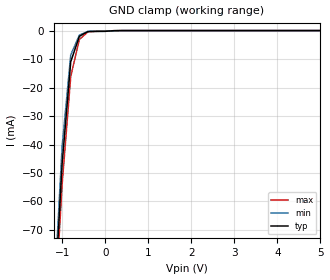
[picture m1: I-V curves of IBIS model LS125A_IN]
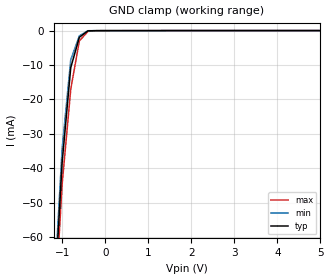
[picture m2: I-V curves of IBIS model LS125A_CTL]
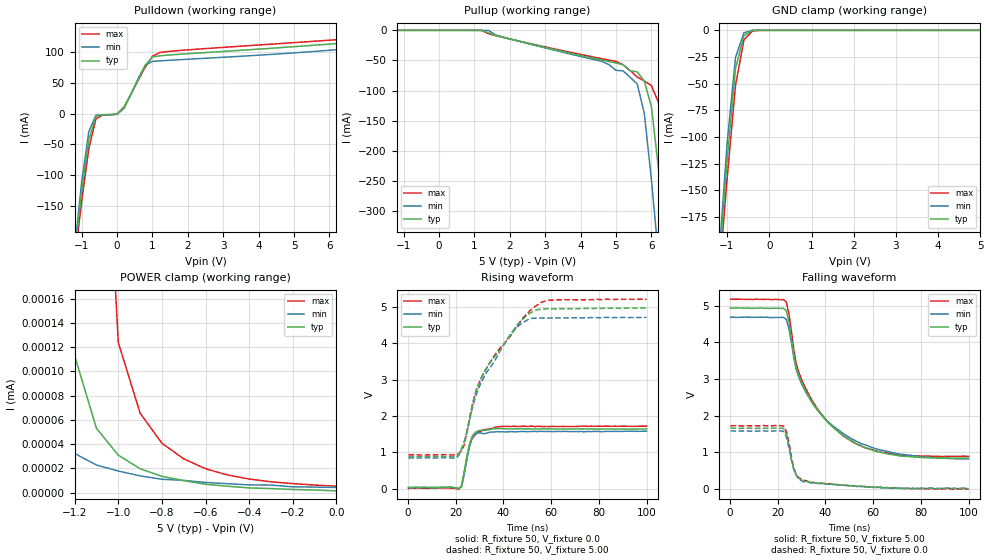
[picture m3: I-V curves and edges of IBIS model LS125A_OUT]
|   TEXAS INSTRUMENTS INCORPORATED
|   Standard Linear and Logic Group
|   IBIS Model of SN74LS125A
|   QUADRUPLE BUS BUFFERS WITH THREE-STATE OUTPUTS
|   SOIC 14-pin(D), SOP 14-pin(NS), PDIP 14-pin(N)
[IBIS Ver]   3.1
[Comment Char]  |_char
[File Name]   sn74ls125a.ibs
[File Rev]   1.1
[Date]   JULY 9, 2004
[Source]   File originated at Texas Instruments, Inc.
[Notes]   - FILE REV HISTORY
   - 1.1 Release IBIS file on 07/10/04
   - All test data contained in this file are derived from
   actual measurements.
   - The measurements used D package.
[Disclaimer] Property of Texas Instruments Incorporated.  Unauthorized
   reproduction and/or distribution is strictly prohibited.
   This product is protected under copyright law.
   Created 2000, (C) Copyright 2000, Texas Instruments Inc.,
   All Rights Reserved.
   UNLESS THERE IS A SIGNED, WRITTEN AGREEMENT TO THE
   CONTRARY, TEXAS INSTRUMENTS () IS PROVIDING THE IBIS
   MODELS  AND WITHOUT ANY WARRANTY, EXPRESSED OR
   IMPLIED.  TI assumes no liability for:
   1) the accuracy of the IBIS models provided to your
   company;
   2) the proper functioning of these IBIS Models in your
   design or for any resulting applications; or
   3) infringement of patents, copyrights or intellectual
   property rights resulting from your use of these IBIS
   models.
   TI provides IBIS Models as a service to our customers.
   You and your company shall not distribute, sell or give
   these models to anyone else without prior written
   permission from TI.
   TI reserves the right to make changes to our products or
   to discontinue any semiconductor product or service
   without notice, and advises our customers to obtain the
   latest version of relevant information to verify, before
   placing orders, that the information being relied on is
   current.
   Please be aware that your receipt and use of the IBIS
   information provided shall serve as acceptance of these
   terms and conditions.  If you do not accept these terms,
   you should return or destroy the IBIS models and any
   other accompanying information immediately.
|   Component LS125A_D
[Component]   LS125A_D
[Manufacturer]  Texas Instruments, Inc.
[Package]
|   typ   min   max
R_pkg   0.039   0.028   0.049
L_pkg   3.453nH   2.350nH   4.375nH
C_pkg   0.521pF   0.254pF   0.708pF
[Pin]   signal_name   model_name   R_pin   L_pin   C_pin
1   1G_BAR   LS125A_CTL   0.042   4.336nH   0.703pF
2   1A   LS125A_IN   0.049   3.778nH   0.634pF
3   1Y   LS125A_OUT   0.028   3.449nH   0.518pF
4   2G_BAR   LS125A_CTL   0.029   2.393nH   0.254pF
5   2A   LS125A_IN   0.028   2.350nH   0.264pF
6   2Y   LS125A_OUT   0.048   3.312nH   0.483pF
7   GND   GND   0.043   3.629nH   0.604pF
8   3Y   LS125A_OUT   0.044   4.375nH   0.708pF
9   3A   LS125A_IN   0.042   4.336nH   0.703pF
10   3G_BAR   LS125A_CTL   0.049   3.778nH   0.634pF
11   4Y   LS125A_OUT   0.028   3.449nH   0.518pF
12   4A   LS125A_IN   0.029   2.393nH   0.255pF
13   4G_BAR   LS125A_CTL   0.028   2.350nH   0.264pF
14   VCC   POWER   0.048   3.312nH   0.483pF
|   Component LS125A_NS
[Component]   LS125A_NS
[Manufacturer]  Texas Instruments, Inc.
[Package]
|   typ   min   max
R_pkg   0.042   0.035   0.049
L_pkg   3.147nH   2.164nH   4.219nH
C_pkg   0.404pF   0.241pF   0.562pF
[Pin]   signal_name   model_name   R_pin   L_pin   C_pin
1   1G_BAR   LS125A_CTL   0.049   4.215nH   0.562pF
2   1A   LS125A_IN   0.046   3.675nH   0.480pF
3   1Y   LS125A_OUT   0.037   2.527nH   0.332pF
4   2G_BAR   LS125A_CTL   0.035   2.164nH   0.241pF
5   2A   LS125A_IN   0.035   2.164nH   0.241pF
6   2Y   LS125A_OUT   0.037   2.527nH   0.332pF
7   GND   GND   0.046   3.675nH   0.480pF
8   3Y   LS125A_OUT   0.049   4.215nH   0.562pF
9   3A   LS125A_IN   0.049   4.219nH   0.562pF
10   3G_BAR   LS125A_CTL   0.046   3.679nH   0.480pF
11   4Y   LS125A_OUT   0.037   2.531nH   0.333pF
12   4A   LS125A_IN   0.035   2.168nH   0.241pF
13   4G_BAR   LS125A_CTL   0.035   2.168nH   0.241pF
14   VCC   POWER   0.037   2.531nH   0.333pF
| Component ls14_N 14-pin PDIP
[Component]   LS125AA_N
[Manufacturer]   Texas Instruments, Inc.
[Package]
|   typ   min   max
R_pkg   4.500e-02   3.700e-02   6.300e-02
L_pkg   5.407e-09   3.922e-09   6.942e-09
C_pkg   3.890e-13   2.050e-13   6.040e-13
[Pin]   signal_name   model_name   R_pin   L_pin   C_pin
1   1G_BAR   LS125A_CTL   6.300e-02   6.942e-09   6.040e-13
2   1A   LS125A_IN   3.700e-02   6.200e-09   4.060e-13
3   1Y   LS125A_OUT   4.200e-02   4.389e-09   3.220e-13
4   2G_BAR   LS125A_CTL   3.800e-02   3.922e-09   2.050e-13
5   2A   LS125A_IN   3.900e-02   4.301e-09   2.980e-13
6   2Y   LS125A_OUT   3.800e-02   5.329e-09   3.560e-13
7   GND   GND   5.300e-02   6.510e-09   5.440e-13
8   3Y   LS125A_OUT   5.300e-02   6.437e-09   5.390e-13
9   3A   LS125A_IN   3.900e-02   5.352e-09   3.470e-13
10   3G_BAR   LS125A_CTL   4.200e-02   4.473e-09   2.970e-13
11   4Y   LS125A_OUT   4.400e-02   4.326e-09   2.250e-13
12   4A   LS125A_IN   4.200e-02   4.295e-09   2.800e-13
13   4G_BAR   LS125A_CTL   4.200e-02   6.318e-09   4.180e-13
14   VCC   POWER   6.100e-02   6.900e-09   6.030e-13
| Models and submodels in the file (3): LS125A_IN (Input), LS125A_CTL (Input), LS125A_OUT (Output)
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|   Model LS125A_IN
[Model]   LS125A_IN
Model_type  Input
Polarity   Non-Inverting
Vinl = 0.8
Vinh = 2.0
| variable   typ   min   max
C_comp   1.35pf   1.01pf   1.69pf
[Temperature Range]   25   0   70
[Voltage Range]   5.00   4.75   5.25
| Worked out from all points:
|   GND clamp passes 1 mA (typ) near -0.48 V on its own axis
[GND Clamp]
|   Voltage   I(typ)   I(min)   I(max)
-5V       -1.507A    -1.589A    -1.376A
-1.2V     -101.1mA   -97.2mA    -106.4mA
-1V       -46.71mA   -40.6mA    -53.99mA
-800mV    -10.94mA   -8.523mA   -16.11mA
-600mV    -2mA       -1.603mA   -3.101mA
-400mV    -325.4uA   -299.5uA   -465.4uA
200mV     -43.97uA   -69.32uA   -26.08uA
5V        4.815nA    2.869nA    16.86nA
|   Model LS125A_CTL
[Model]   LS125A_CTL
Model_type  Input
Polarity   Inverting
Vinl = 0.8
Vinh = 2.0
| variable   typ   min   max
C_comp   1.35pf   1.01pf   1.69pf
[Temperature Range]   25   0   70
[Voltage Range]   5.00   4.75   5.25
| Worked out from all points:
|   GND clamp passes 1 mA (typ) near -0.50 V on its own axis
[GND Clamp]
|   Voltage   I(typ)   I(min)   I(max)
-5V       -1.311A    -1.374A    -1.202A
-1.2V     -82.87mA   -79.26mA   -87.87mA
-1V       -38.39mA   -34.34mA   -44.72mA
-800mV    -10.77mA   -8.506mA   -17.06mA
-600mV    -1.955mA   -1.528mA   -3.015mA
-400mV    -71.82uA   -40.41uA   -243uA
-200mV    -23.98uA   -25.02uA   -22.13uA
5V        1.516nA    544.1pA    4.133nA
|   Model LS125A_OUT
[Model]   LS125A_OUT
Model_type  Output
Polarity   Non-Inverting
Vmeas = 1.3v
Cref = 45pf
Rref = 667
Vref = 0
| variable   typ   min   max
C_comp   5.60pf   4.20pf   7.00pf
[Temperature Range]   25   0   70
[Voltage Range]   5.00   4.75   5.25
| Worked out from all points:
|   slope of the pulldown table from 0 to 0.75 V, typ, clamps not added: 10.2 ohm
|   GND clamp passes 1 mA (typ) near -0.44 V on its own axis
|   rising waveform, R_fixture 50, V_fixture 0.0: 20-80 % time 3.01ns typ, 2.92ns min, 3.61ns max; typ from 0.03 V to 1.65 V
|   falling waveform, R_fixture 50, V_fixture 5.00: 20-80 % time 17.9ns typ, 19.9ns min, 16.6ns max; typ from 4.93 V to 0.845 V
|   rising waveform, R_fixture 50, V_fixture 5.00: 20-80 % time 16.9ns typ, 15ns min, 19.1ns max; typ from 0.878 V to 4.98 V
|   falling waveform, R_fixture 50, V_fixture 0.0: 20-80 % time 4.02ns typ, 3.99ns min, 4.07ns max; typ from 1.66 V to 0.01 V
[Pulldown]
|   Voltage   I(typ)   I(min)   I(max)
-5V       -2.251A    -2.394A    -2.101A
-1.2V     -228.3mA   -218.6mA   -236.3mA
-1V       -125.8mA   -109.7mA   -141.3mA
-800mV    -43.31mA   -29.43mA   -57.06mA
-600mV    -4.546mA   -2.797mA   -8.615mA
0V        -1.168mA   -1.308mA   -1.051mA
200mV     10.18mA    8.496mA    11.05mA
800mV     78.07mA    78.39mA    75.4mA
1V        91.36mA    84.23mA    92.47mA
1.4V      94.2mA     85.75mA    99.96mA
5.6V      110.5mA    100.4mA    116.9mA
10V       131.3mA    124.3mA    139.6mA
[Pullup]
|   Voltage   I(typ)   I(min)   I(max)
-5V       2.11uA     674.1nA    5.805uA
1.4V      -4.41mA    -283.6uA   -5.664mA
4.6V      -49.31mA   -51.51mA   -47.11mA
5V        -54.19mA   -66.44mA   -51.67mA
5.2V      -56.96mA   -67.32mA   -57.4mA
5.6V      -68.94mA   -89.12mA   -77.47mA
5.8V      -84.15mA   -137.7mA   -84.06mA
6V        -126.8mA   -247.3mA   -91.78mA
6.2V      -228.9mA   -374.8mA   -119.5mA
6.4V      -345.4mA   -478.1mA   -213.4mA
6.6V      -442.7mA   -589.6mA   -319.5mA
10V       -2.246A    -2.52A     -1.968A
[GND Clamp]
|   Voltage   I(typ)   I(min)   I(max)
-5V       -2.246A    -2.38A     -2.092A
-1.2V     -227.1mA   -217.8mA   -235.5mA
-1V       -122.7mA   -106.5mA   -139.6mA
-800mV    -35.85mA   -25.45mA   -51.61mA
-600mV    -4.91mA    -2.303mA   -8.973mA
-400mV    -82.58uA   -8.365uA   -568.8uA
-200mV    -132.2nA   -15.39nA   -2.507uA
5V        1.388nA    5.348nA    3.84nA
[POWER Clamp]
|   Voltage   I(typ)   I(min)   I(max)
-5V       197.2uA    217.1uA    183.8uA
-1.5V     16.97uA    8.357uA    23.31uA
-1.4V     11.66uA    126nA      18.74uA
-1.3V     2.163uA    52.81nA    14.14uA
-1.2V     113nA      32.27nA    9.032uA
-1.1V     53nA       22.72nA    460.4nA
-1V       30.87nA    17.79nA    124nA
-900mV    19.67nA    13.77nA    65.57nA
-800mV    13.4nA     10.96nA    40.71nA
-700mV    9.873nA    10.04nA    27.81nA
-500mV    5.229nA    7.333nA    14.52nA
9.77fV    1.388nA    4.194nA    5.241nA
[Ramp]
| variable   typ   min   max
dV/dt_r   9.900E-01/2.990E-09   9.400E-01/2.750E-09   1.040E+00/3.610E-09
dV/dt_f   2.510E+00/1.821E-08   2.370E+00/2.021E-08   2.630E+00/1.697E-08
R_load = 50
[Rising Waveform]
R_fixture = 50
V_fixture = 0.0
V_fixture_min = 0.0
V_fixture_max = 0.0
C_fixture = 0pf
L_fixture = 0nH
|   Time   V(typ)   V(min)   V(max)
195.3ps   29.79mV    34.4mV     6.6mV
21.29ns   6.75mV     6.45mV     -12.32mV
22.46ns   85.9mV     55.9mV     80.1mV
24.8ns    942mV      854.1mV    904.9mV
25.78ns   1.23V      1.163V     1.173V
26.76ns   1.426V     1.384V     1.367V
27.73ns   1.523V     1.488V     1.456V
29.69ns   1.601V     1.536V     1.563V
39.45ns   1.651V     1.57V      1.717V
100ns     1.646V     1.585V     1.72V
[Falling Waveform]
R_fixture = 50
V_fixture = 5.00
V_fixture_min = 4.75
V_fixture_max = 5.25
C_fixture = 0pf
L_fixture = 0nH
|   Time   V(typ)   V(min)   V(max)
195.3ps   4.93V      4.684V     5.17V
23.63ns   4.85V      4.619V     5.091V
24.8ns    4.527V     4.331V     4.733V
26.76ns   3.653V     3.563V     3.778V
27.73ns   3.319V     3.262V     3.424V
30.66ns   2.815V     2.774V     2.884V
39.45ns   1.925V     1.945V     1.949V
49.22ns   1.38V      1.437V     1.371V
66.8ns    944.4mV    1.012V     969.4mV
100ns     845.2mV    818.5mV    887.6mV
[Rising Waveform]
R_fixture = 50
V_fixture = 5.00
V_fixture_min = 4.75
V_fixture_max = 5.25
C_fixture = 0pf
L_fixture = 0nH
|   Time   V(typ)   V(min)   V(max)
195.3ps   878.3mV    843.7mV    933.9mV
20.12ns   889.1mV    845.5mV    935.7mV
22.46ns   1.072V     1.112V     1.055V
23.63ns   1.268V     1.32V      1.214V
27.73ns   2.506V     2.413V     2.512V
30.66ns   3.043V     2.923V     3.056V
42.38ns   4.198V     4.187V     4.156V
48.24ns   4.677V     4.577V     4.703V
58.98ns   4.964V     4.695V     5.187V
100ns     4.977V     4.716V     5.212V
[Falling Waveform]
R_fixture = 50
V_fixture = 0.0
V_fixture_min = 0.0
V_fixture_max = 0.0
C_fixture = 0pf
L_fixture = 0nH
|   Time   V(typ)   V(min)   V(max)
195.3ps   1.66V      1.581V     1.721V
22.46ns   1.65V      1.573V     1.718V
23.63ns   1.489V     1.417V     1.564V
24.8ns    1.144V     1.096V     1.232V
25.78ns   784.5mV    773.1mV    852mV
26.76ns   538.7mV    526.5mV    561.9mV
28.71ns   296.5mV    278.1mV    315.6mV
30.66ns   224.8mV    203mV      239.8mV
60.94ns   47.2mV     40.9mV     44mV
100ns     10.42mV    22.32mV    950uV
